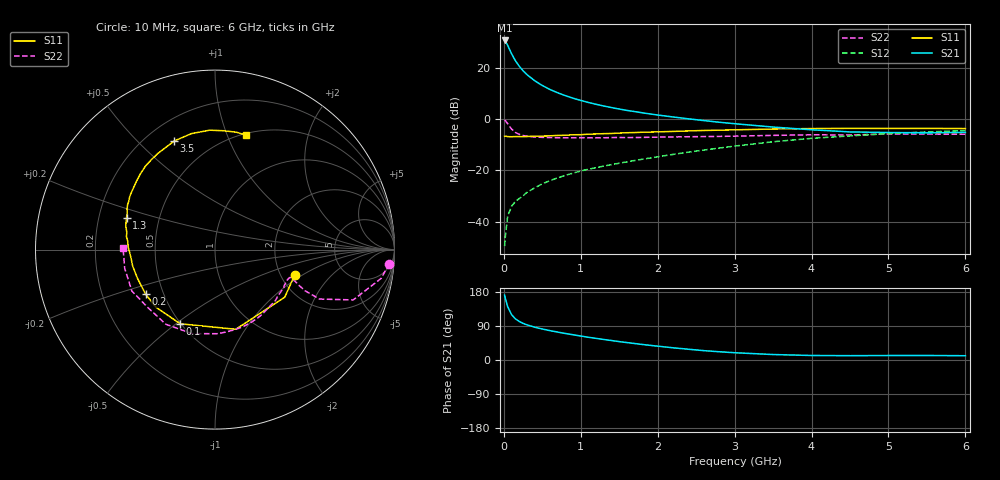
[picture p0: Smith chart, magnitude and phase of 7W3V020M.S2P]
! Infineon Technologies  Discrete & RF Semiconductors
! BFS17W
! Si NPN RF Bipolar Junction Transistor in SOT323
! VCE = 3 V  IC = 20 mA
! Common Emitter S-Parameters:  August  1999
# GHz  S  MA  R  50
!  f  S11  S21  S12  S22
! GHz  MAG  ANG  MAG  ANG  MAG  ANG  MAG  ANG
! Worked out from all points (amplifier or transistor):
!   36 points, 10 MHz to 6 GHz, reference 50 ohm
!   highest |S21| = 30.9 dB at 10 MHz (marker M1)
!   |S21| within 3 dB of that: start of sweep to 66.64 MHz
!   unconditionally stable (mu >= 1): 246.5 MHz to 2.357 GHz; 4.456 GHz to end of sweep
!   at 250 MHz: K = 1.01, MAG = 23.9 dB, |S12| = -29.9 dB
!   at 1.4 GHz: K = 1.20, MAG = 8.5 dB, |S12| = -17.7 dB
!   at 6 GHz: K = 1.07, MAG = -2.0 dB, |S12| = -4.4 dB
!   S11 on the Smith chart (normalised r, x): 10 MHz: 2.38, -0.85; 100 MHz: 0.50, -0.52; 200 MHz: 0.40, -0.25; 1.3 GHz: 0.32, +0.16; 3.5 GHz: 0.31, +0.65; 6 GHz: 0.52, +1.17
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0.01  0.4659 -17.5  34.92 171.2  0.0033 80.8  0.9734 -4.6
0.02  0.4704 -34.3  34.01 162.1  0.0052 81.2  0.94 -9.8
0.05  0.4587 -75.4  28.02 140.6  0.0128 66.8  0.8195 -20.0
0.1  0.4564 -115.1  19.24 119.9  0.0199 57.7  0.6449 -25.3
0.15  0.4597 -135.6  14.05 108.6  0.0246 57.6  0.553 -24.6
0.2  0.4595 -147.2  10.96 101.7  0.0282 60.7  0.5092 -23.1
0.25  0.4578 -154.9  8.92 96.7  0.0319 61.7  0.4822 -21.7
0.3  0.461 -160.3  7.515 92.8  0.0372 63.3  0.4685 -20.9
0.4  0.468 -168.9  5.706 86.6  0.0455 65.9  0.4505 -20.3
0.5  0.4698 -174.1  4.589 81.8  0.0547 67.8  0.4443 -20.5
0.6  0.4761 -178.2  3.83 77.5  0.0633 68.5  0.44 -21.5
0.7  0.4843 178.2  3.306 73.6  0.0718 68.8  0.4368 -23.1
0.9  0.4989 171.6  2.589 66.6  0.0885 69.9  0.4344 -26.9
1.1  0.5123 165.7  2.138 60.0  0.1059 70.1  0.436 -31.5
1.3  0.5243 160.1  1.823 54.1  0.122 70.3  0.4355 -36.9
1.7  0.5509 150.7  1.419 43.5  0.1566 70.7  0.4405 -48.0
2.2  0.5799 139.0  1.112 32.2  0.2059 70.3  0.4524 -63.3
2.8  0.6135 125.3  0.878 21.8  0.274 67.1  0.4636 -82.6
3.5  0.6465 110.6  0.706 14.4  0.3638 60.7  0.4853 -105.4
4.5  0.666 92.6  0.567 11.4  0.4738 47.6  0.4941 -139.3
5.5  0.6648 79.6  0.545 11.9  0.566 34.9  0.5138 -168.3
6  0.6598 74.6  0.556 11.3  0.602 28.8  0.5121 179.0
